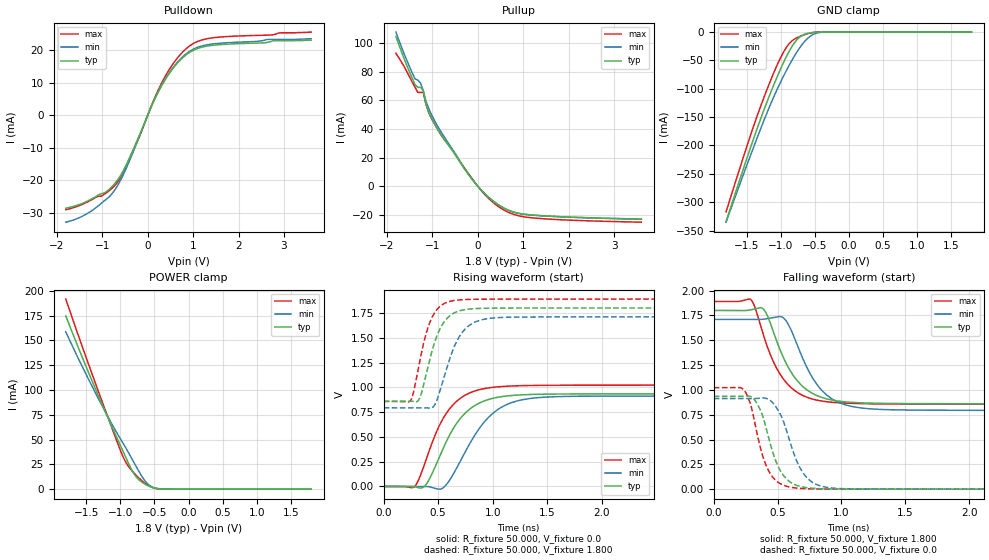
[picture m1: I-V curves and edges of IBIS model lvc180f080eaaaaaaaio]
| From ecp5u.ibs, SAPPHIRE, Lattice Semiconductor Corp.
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|   Model lvc180f080eaaaaaaaio
[Model] lvc180f080eaaaaaaaio
Model_type I/O
Polarity   Non-Inverting
Enable   Active-Low
Vinl =  0.630V
Vinh =  1.170V
Vmeas =  0.900V
Cref =  0.0F
Rref =  1.000M
Vref =  0.0V
C_comp   5.000pF   4.000pF   5.500pF
[Temperature Range]   25.000   0.125k   -40.000
[Voltage Range]   1.800V   1.710V   1.890V
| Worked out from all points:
|   slope of the pulldown table from 0 to 0.27 V, typ, clamps not added: 33.1 ohm
|   slope of the pullup table from 0 to 0.27 V, typ, clamps not added: 31.2 ohm
|   GND clamp passes 1 mA (typ) near -0.54 V on its own axis
|   POWER clamp passes 1 mA (typ) near -0.49 V on its own axis
|   rising waveform, R_fixture 50.000, V_fixture 0.0: 20-80 % time 287ps typ, 325ps min, 263ps max; typ from 0 V to 0.934 V
|   rising waveform, R_fixture 50.000, V_fixture 1.800: 20-80 % time 156ps typ, 184ps min, 139ps max; typ from 0.86 V to 1.8 V
|   falling waveform, R_fixture 50.000, V_fixture 1.800: 20-80 % time 226ps typ, 229ps min, 216ps max; typ from 1.8 V to 0.86 V
|   falling waveform, R_fixture 50.000, V_fixture 0.0: 20-80 % time 141ps typ, 160ps min, 126ps max; typ from 0.934 V to 0 V
[Pulldown]
|Voltage   I(typ)   I(min)   I(max)
-1.8V     -28.53mA   -32.84mA   -29.01mA
-1.2V     -25.46mA   -29.03mA   -25.7mA
-900mV    -23.35mA   -25.68mA   -23.75mA
-660mV    -19.84mA   -21.55mA   -20.51mA
-420mV    -13.7mA    -14.59mA   -14.42mA
60mV      2.026mA    2.064mA    2.192mA
240mV     7.384mA    7.52mA     8.023mA
540mV     14.17mA    14.41mA    15.5mA
840mV     18.59mA    18.89mA    20.45mA
1.08V     20.52mA    20.88mA    22.66mA
1.44V     21.61mA    22.02mA    23.91mA
3.6V      23.2mA     23.62mA    25.66mA
[Pullup]
|Voltage   I(typ)   I(min)   I(max)
-1.8V     104.5mA    107.6mA    92.84mA
-1.38V    70.9mA     74.9mA     69.09mA
-1.26V    68.99mA    72.12mA    65.48mA
-1.2V     66.93mA    66.81mA    65.48mA
-1.14V    57.38mA    59.48mA    57.36mA
-1.08V    51.83mA    54.35mA    51.48mA
-900mV    40.67mA    42.94mA    40.69mA
-180mV    7.161mA    7.234mA    7.646mA
360mV     -10.95mA   -10.92mA   -11.94mA
720mV     -17.31mA   -17.4mA    -18.86mA
1.08V     -19.76mA   -19.89mA   -21.68mA
3.6V      -22.97mA   -23.08mA   -25.16mA
[GND_clamp]
|Voltage   I(typ)   I(min)   I(max)
-1.8V     -334.4mA   -335.3mA   -317.1mA
-1.4V     -189.3mA   -204.4mA   -167.3mA
-1.28V    -148.9mA   -166.7mA   -126.7mA
-1.12V    -99.04mA   -119.7mA   -77.45mA
-1V       -64.9mA    -88.2mA    -45.18mA
-920mV    -44.4mA    -68.92mA   -27.88mA
-840mV    -26.71mA   -51.09mA   -16.18mA
-720mV    -8.754mA   -27.82mA   -7.821mA
-640mV    -3.53mA    -15.52mA   -4.188mA
-560mV    -1.27mA    -6.791mA   -1.597mA
-400mV    -49.63uA   -425.4uA   -44.12uA
1.8V      0A         0A         0A
[POWER_clamp]
|Voltage   I(typ)   I(min)   I(max)
-1.8V     174.6mA    158.5mA    191.6mA
-1.36V    100.3mA    96.28mA    105.7mA
-1.12V    62.39mA    65.2mA     61.09mA
-960mV    38.11mA    46.28mA    32.52mA
-880mV    25.96mA    36.75mA    22.79mA
-800mV    15.45mA    26.86mA    16.3mA
-720mV    9.004mA    17.05mA    10.75mA
-640mV    5.132mA    8.487mA    6.134mA
-560mV    2.382mA    3.217mA    2.693mA
-520mV    1.425mA    1.849mA    1.506mA
-360mV    88.16uA    177.6uA    42.1uA
1.8V      0A         0A         0A
[Ramp]
| variable   typ   min   max
dV/dt_r 0.561/0.291n   0.547/0.327n   0.613/0.263n
dV/dt_f 0.564/0.229n   0.550/0.235n   0.620/0.219n
R_load = 50.000
[Rising Waveform]
R_fixture= 50.000
V_fixture= 0.0
V_fixture_min= 0.0
V_fixture_max= 0.0
|time   V(typ)   V(min)   V(max)
0s        0V         0V         0V
292ps     -4.859mV   -190.7uV   9.257mV
392ps     24.05mV    -902.6uV   278.5mV
545ps     382.1mV    -14.42mV   684.5mV
755ps     747mV      362.5mV    925mV
898ps     851.4mV    615.8mV    981.2mV
1.035ns   896.9mV    766.4mV    1.003V
1.278ns   924.8mV    875.7mV    1.017V
1.714ns   933mV      908.8mV    1.021V
10ns      934.5mV    912.4mV    1.022V
[Rising Waveform]
R_fixture= 50.000
V_fixture= 1.800
V_fixture_min= 1.710
V_fixture_max= 1.890
|time   V(typ)   V(min)   V(max)
0s        860mV      793.1mV    857.1mV
250ps     859.1mV    793.1mV    870.8mV
329ps     887mV      792.7mV    1.252V
390ps     1.132V     792.2mV    1.545V
450ps     1.391V     798.8mV    1.719V
553ps     1.657V     1.099V     1.844V
690ps     1.77V      1.504V     1.881V
858ps     1.795V     1.667V     1.888V
1.167ns   1.799V     1.707V     1.89V
10ns      1.8V       1.71V      1.89V
[Falling Waveform]
R_fixture= 50.000
V_fixture= 1.800
V_fixture_min= 1.710
V_fixture_max= 1.890
|time   V(typ)   V(min)   V(max)
0s        1.8V       1.71V      1.89V
292ps     1.806V     1.71V      1.907V
395ps     1.805V     1.713V     1.527V
544ps     1.328V     1.726V     1.111V
707ps     1.023V     1.287V     937.4mV
817ps     937.5mV    1.039V     894.1mV
939ps     894.3mV    899.3mV    873.5mV
1.147ns   869.4mV    818.9mV    861.9mV
1.549ns   861.6mV    796.5mV    858.4mV
10ns      860mV      793.1mV    857.1mV
[Falling Waveform]
R_fixture= 50.000
V_fixture= 0.0
V_fixture_min= 0.0
V_fixture_max= 0.0
|time   V(typ)   V(min)   V(max)
0s        934.5mV    912.4mV    1.022V
246ps     936.4mV    912.5mV    981.7mV
292ps     930.1mV    911.7mV    837.4mV
351ps     834mV      915.7mV    490mV
447ps     434.7mV    888.5mV    147.5mV
537ps     154.2mV    710.3mV    44.54mV
666ps     30.97mV    238.6mV    8.952mV
805ps     6.529mV    46.85mV    2.04mV
1.063ns   904.5uV    3.25mV     294.1uV
10ns      0V         0V         0V
